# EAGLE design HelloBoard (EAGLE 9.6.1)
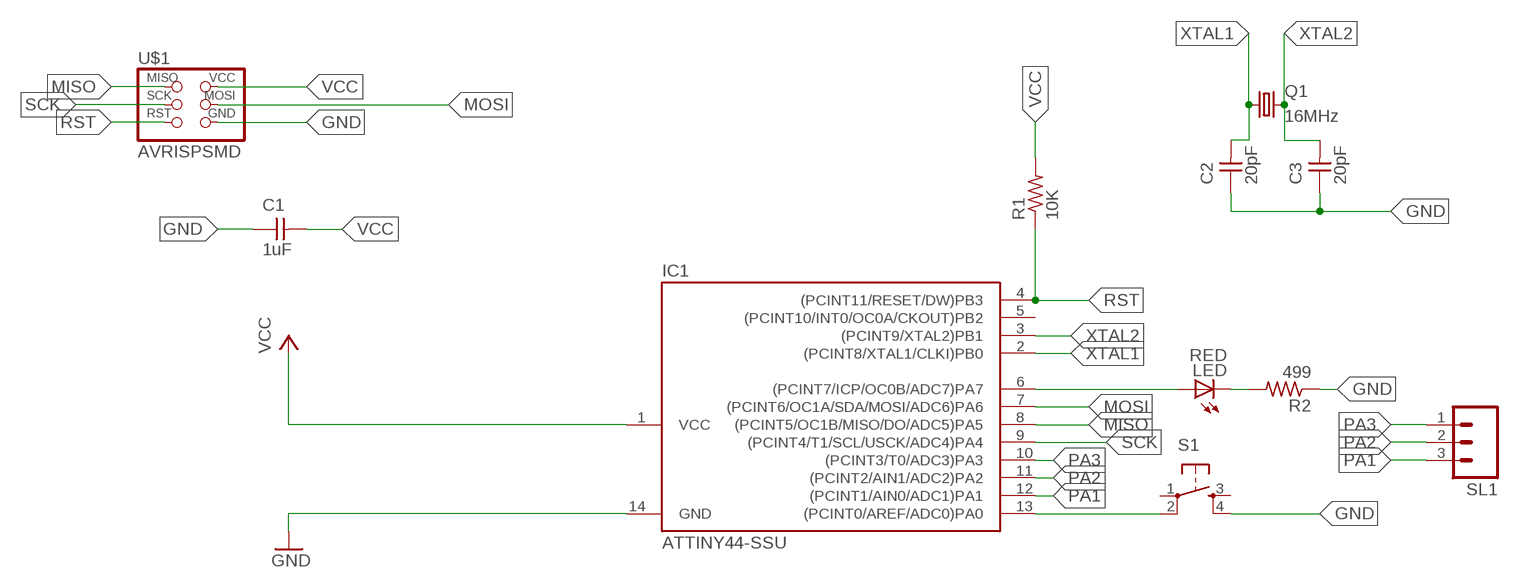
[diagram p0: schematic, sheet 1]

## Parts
C1  1uF  UNPOLARIZED_CAPACITOR1206  [1206]
C2  20pF  UNPOLARIZED_CAPACITOR1206  [1206]
C3  20pF  UNPOLARIZED_CAPACITOR1206  [1206]
IC1  ATTINY44-SSU  [SOIC14]
LED  RED  LED1206  [1206]
Q1  16MHz  CSM-7X-DU  [CSM-7X-DU]
R1  10K  RESISTOR1206  [1206]
R2  499  RESISTOR1206  [1206]
S1  6MM_SWITCH6MM_SWITCH  [6MM_SWITCH]
SL1  M03  [03P]
U$1  AVRISPSMD  [2X03SMD]

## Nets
GND: C1.1 C2.1 C3.1 IC1.14(GND) R2.1 S1.4(S1) U$1.6(GND)
MISO: IC1.8((PCINT5/OC1B/MISO/DO/ADC5)PA5) U$1.1(MISO)
MOSI: IC1.7((PCINT6/OC1A/SDA/MOSI/ADC6)PA6) U$1.4(MOSI)
N$1: IC1.6((PCINT7/ICP/OC0B/ADC7)PA7) LED.1(A)
N$2: LED.2(C) R2.2
N$3: IC1.13((PCINT0/AREF/ADC0)PA0) S1.2(P1)
PA1: IC1.12((PCINT1/AIN0/ADC1)PA1) SL1.3
PA2: IC1.11((PCINT2/AIN1/ADC2)PA2) SL1.2
PA3: IC1.10((PCINT3/T0/ADC3)PA3) SL1.1
RST: IC1.4((PCINT11/RESET/DW)PB3) R1.1 U$1.5(RST)
SCK: IC1.9((PCINT4/T1/SCL/USCK/ADC4)PA4) U$1.3(SCK)
VCC: C1.2 IC1.1(VCC) R1.2 U$1.2(VCC)
XTAL1: C2.2 IC1.2((PCINT8/XTAL1/CLKI)PB0) Q1.1
XTAL2: C3.2 IC1.3((PCINT9/XTAL2)PB1) Q1.2
Unconnected: IC1.5((PCINT10/INT0/OC0A/CKOUT)PB2) S1.1(P) S1.3(S)

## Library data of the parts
C1-C3 = FAB_Hello:UNPOLARIZED_CAPACITOR: unpolarized_capacitor
IC1 = FAB_Hello:ATTINY44
LED = FAB_Hello:LED
Q1 = FAB_Hello:CSM-7X-DU: SMD CRYSTAL; OC_FARNELL: unknown; OC_NEWARK: unknown
R1 R2 = FAB_Hello:RESISTOR
S1 = FAB_Hello:6MM_SWITCH: OMRON SWITCH
SL1 = con-amp-quick:M03: AMP QUICK CONNECTOR; OC_FARNELL: unknown; OC_NEWARK: unknown
U$1 = FAB_Hello:AVRISP

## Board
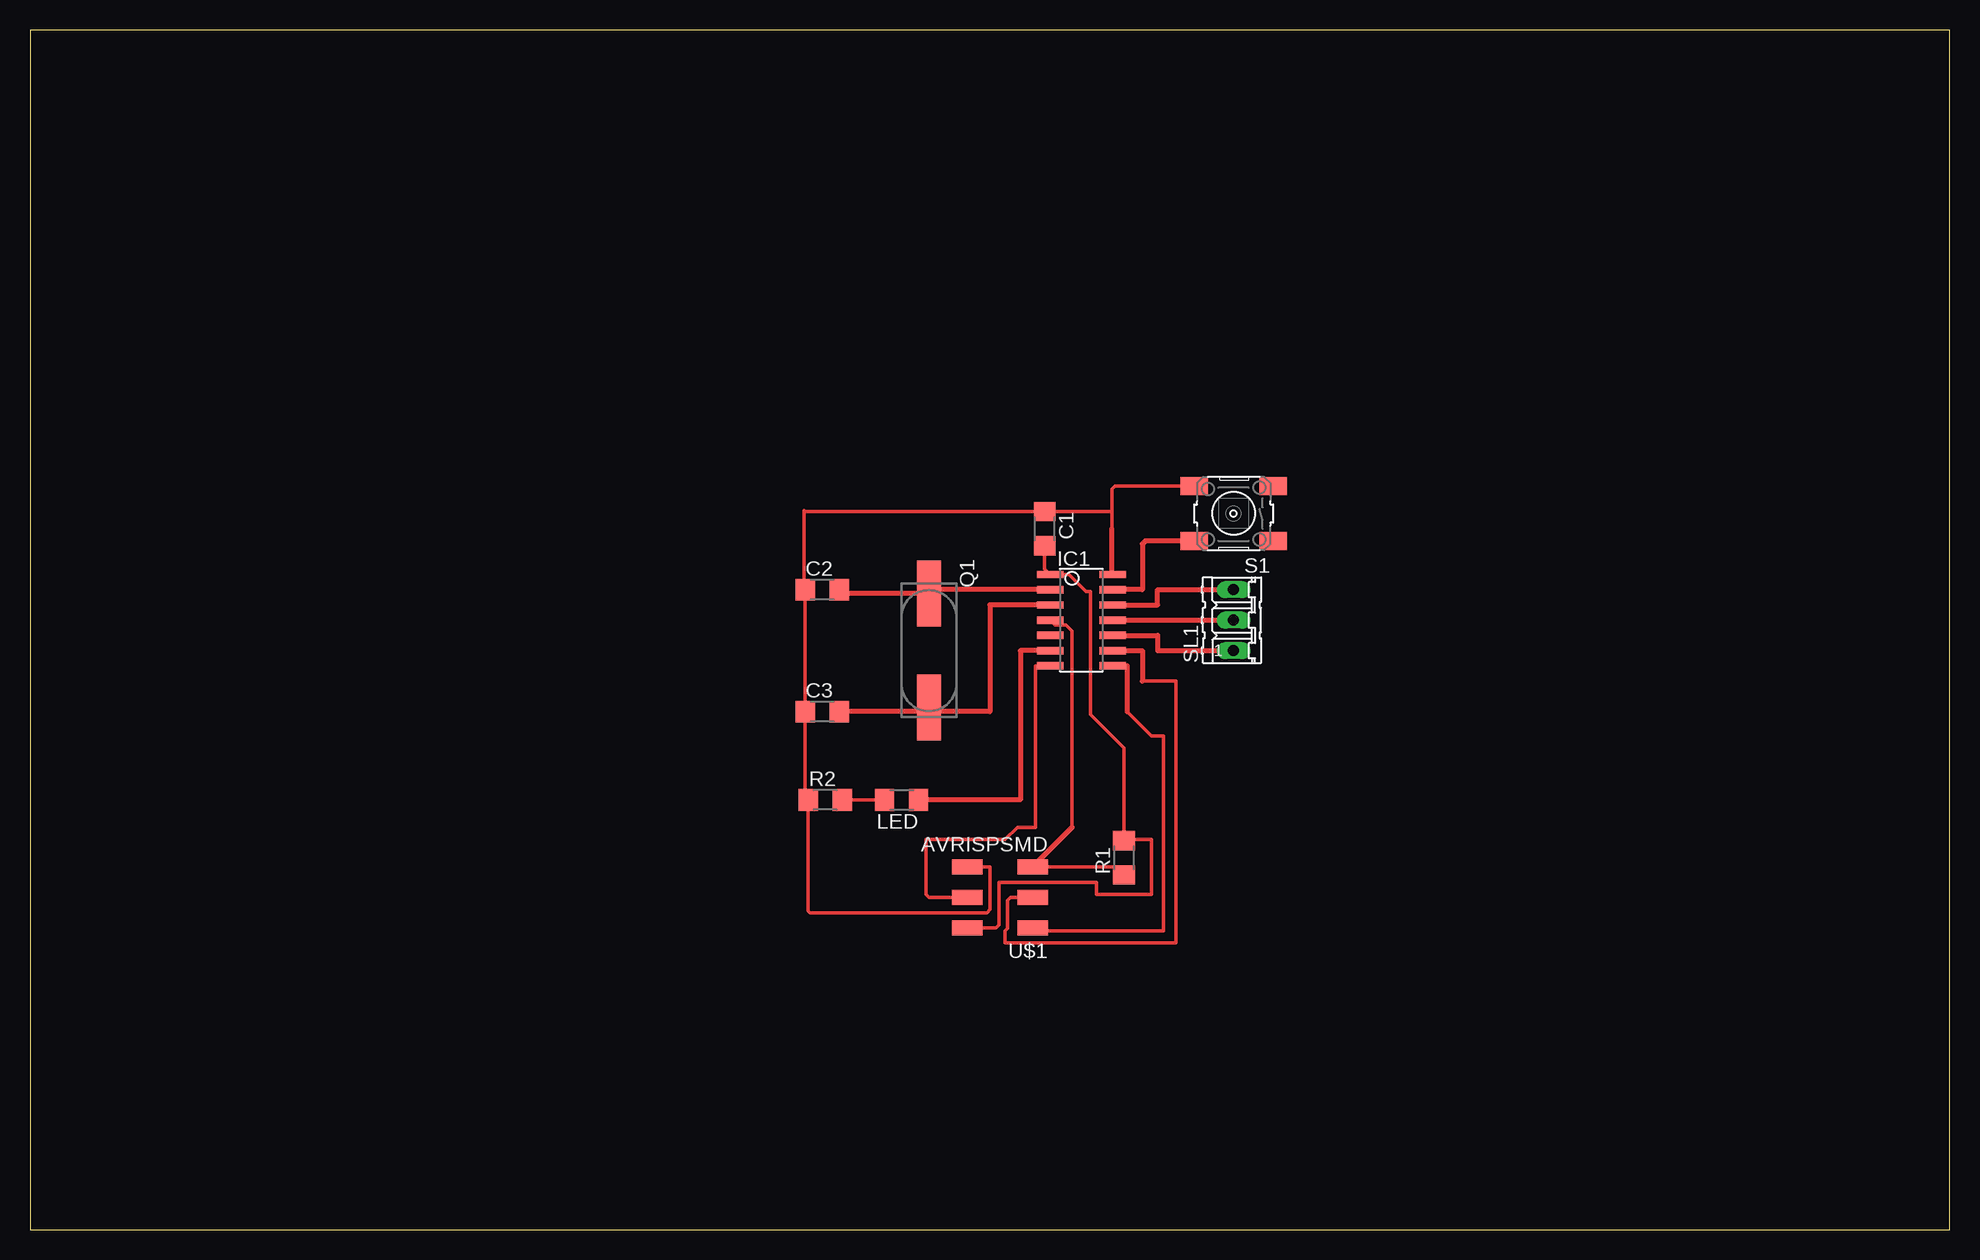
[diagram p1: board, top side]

Size 160 x 100 mm. Coordinates in mm from the lower left corner, seen from the top.
Outline: 0,0 160,0 160,100 0,100 0,0
Copper layers (1*16): Top 0.035mm / dielectric 1.5mm / Bottom 0.035mm
Design rules "default *": minimum track width 6mil, minimum drill 0.35mm, track to track 16mil, track to pad 16mil, pad to pad 16mil, via to via 16mil, smd to smd 16mil, copper to edge 40mil, drill to drill 6mil, minimum pad ring 10mil, minimum via ring 8mil, stop-mask expansion 4mil, vias tented up to drill 0mil, thermal gap 10mil

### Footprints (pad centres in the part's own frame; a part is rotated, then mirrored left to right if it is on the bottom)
1206 = smd 1.6 x 1.803: 1 -1.422,0; 2 1.422,0
SOIC14 = smd 0.61 x 2.21: 1 -3.81,-2.603; 2 -2.54,-2.603; 3 -1.27,-2.603; 4 0,-2.603; 5 1.27,-2.603; 6 2.54,-2.603; 7 3.81,-2.603; 8 3.81,2.603; 9 2.54,2.603; 10 1.27,2.603; 11 0,2.603; 12 -1.27,2.603; 13 -2.54,2.603; 14 -3.81,2.603
CSM-7X-DU = smd 5.5 x 2: 1 -4.75,0; 2 4.75,0
6MM_SWITCH = smd 2.286 x 1.524: 1 -3.302,2.286; 2 3.302,2.286; 3 -3.302,-2.286; 4 3.302,-2.286
03P = drill 0.914 long: 1 -2.54,0; 2 0,0; 3 2.54,0
2X03SMD = smd 2.54 x 1.27: 1 -2.54,2.54; 2 2.92,2.54; 3 -2.54,0; 4 2.92,0; 5 -2.54,-2.54; 6 2.92,-2.54

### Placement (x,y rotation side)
C1  84.58,58.42 270 top
C2  66.04,53.34 0 top
C3  66.04,43.18 0 top
IC1  87.63,50.8 270 top
LED  72.64,35.81 180 top
Q1  74.93,48.26 270 top
R1  91.19,30.99 90 top
R2  66.29,35.81 0 top
S1  100.33,59.69 180 top
SL1  100.33,50.8 90 top
U$1  81.03,27.69 180 top

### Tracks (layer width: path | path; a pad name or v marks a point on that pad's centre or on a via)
GND
  Top 0.305: 90.17,58.42 90.17,59.84 | 90.17,59.84 C1.1 64.62,59.84 64.52,59.94 64.52,53.44 C2.1 C3.1 64.62,36.07 R2.1 64.87,26.57 65.02,26.42 69.09,26.42 | 90.17,59.84 90.17,61.72 90.42,61.98 S1.4 | 69.09,26.42 74.68,26.42 79.76,26.42 80.01,26.67 80.01,30.23 U$1.6 | 69.09,26.42
  Top 0.406: 90.17,58.42 90.17,54.67 IC1.14
MISO
  Top 0.305: 91.44,43.18 93.47,41.15 94.49,41.15 94.49,24.89 83.82,24.89 U$1.1
  Top 0.406: IC1.8 91.44,46.99 91.44,43.18
MOSI
  Top 0.305: IC1.7 83.82,46.99 83.82,33.53 82.3,33.53 81.28,32.51 78.23,32.51 74.68,32.51 74.68,27.94 74.93,27.69 U$1.4
N$1
  Top 0.406: IC1.6 82.55,48.26 82.55,35.81 LED.1
N$2
  Top 0.305: R2.2 LED.2
N$3
  Top 0.406: S1.2 92.96,57.4 92.71,57.15 92.71,53.34 IC1.13
PA1
  Top 0.406: IC1.12 93.98,52.07 93.98,53.34 SL1.3
PA2
  Top 0.406: IC1.11 SL1.2
PA3
  Top 0.406: IC1.10 93.98,49.53 93.98,48.26 SL1.1
RST
  Top 0.305: U$1.5 90.53,30.23 R1.1 | IC1.4 85.43,50.39 86.36,50.39 86.87,49.89 86.87,33.53
  Top 0.406: 86.87,33.53 U$1.5
SCK
  Top 0.305: 92.71,45.72 95.5,45.72 95.5,23.88 81.28,23.88 81.28,24.9 81.48,25.11 81.48,27.43 81.74,27.69 U$1.3
  Top 0.406: IC1.9 92.71,48.26 92.71,45.72
VCC
  Top 0.305: U$1.2 80.52,25.15 80.77,25.4 80.77,28.96 88.9,28.96 88.9,27.94 93.47,27.94 93.47,32.51 91.29,32.51 R1.2 91.19,40.13 88.39,42.93 88.39,53.19 88.04,53.19 86.61,54.61 IC1.1 84.58,55.05 C1.2
XTAL1
  Top 0.406: IC1.2 75.26,53.34 Q1.1 67.79,53.01 C2.2
XTAL2
  Top 0.406: C3.2 74.6,43.18 Q1.2 75.26,43.18 80.01,43.18 80.01,52.07 IC1.3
